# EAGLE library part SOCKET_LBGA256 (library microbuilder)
LBGA256 socket ... pitch is 1 mm
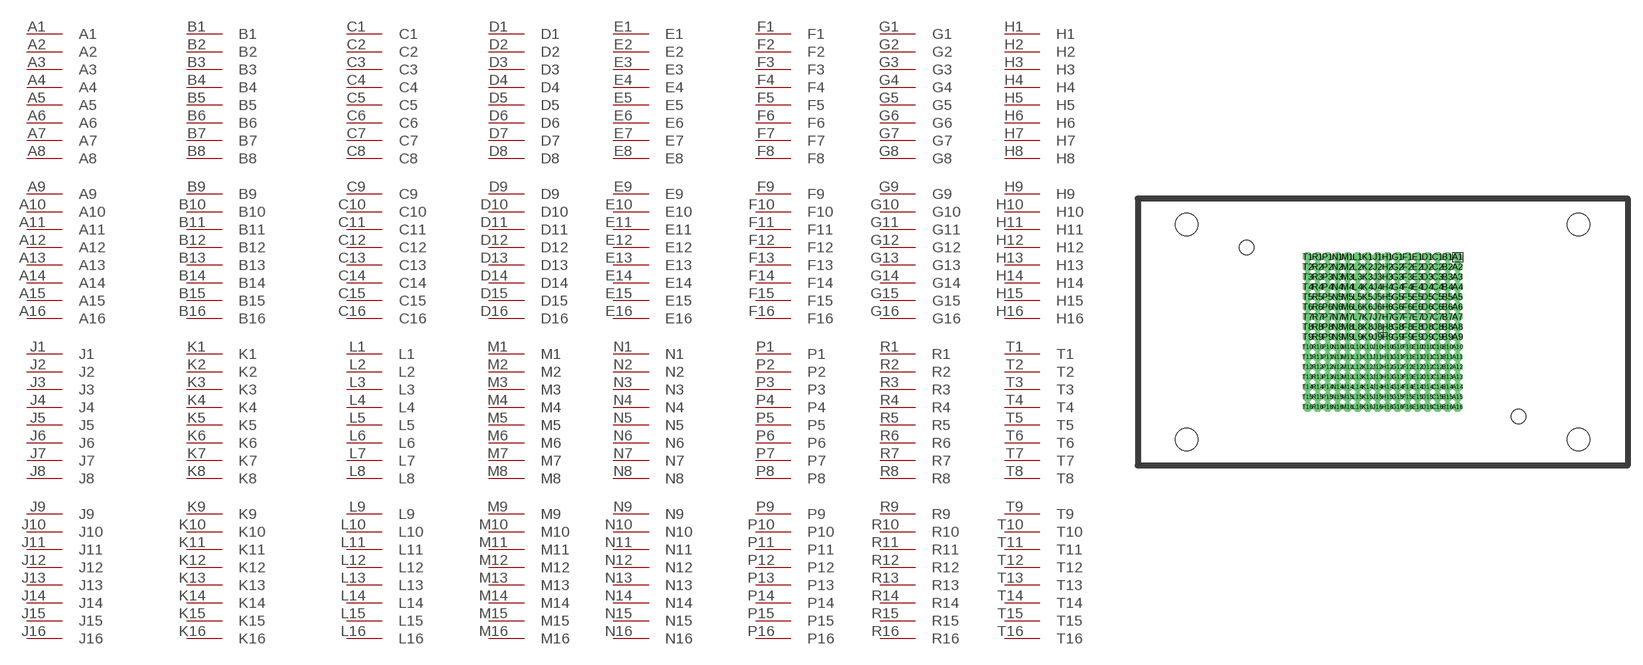
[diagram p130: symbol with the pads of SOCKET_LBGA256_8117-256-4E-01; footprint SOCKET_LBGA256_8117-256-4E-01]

Designator prefix IC

## SOCKET_LBGA256  [SOCKET_LBGA256_8117-256-4E-01]
A1  A1
A2  A2
A3  A3
A4  A4
A5  A5
A6  A6
A7  A7
A8  A8
A9  A9
A10  A10
A11  A11
A12  A12
A13  A13
A14  A14
A15  A15
A16  A16
B1  B1
B2  B2
B3  B3
B4  B4
B5  B5
B6  B6
B7  B7
B8  B8
B9  B9
B10  B10
B11  B11
B12  B12
B13  B13
B14  B14
B15  B15
B16  B16
C1  C1
C2  C2
C3  C3
C4  C4
C5  C5
C6  C6
C7  C7
C8  C8
C9  C9
C10  C10
C11  C11
C12  C12
C13  C13
C14  C14
C15  C15
C16  C16
D1  D1
D2  D2
D3  D3
D4  D4
D5  D5
D6  D6
D7  D7
D8  D8
D9  D9
D10  D10
D11  D11
D12  D12
D13  D13
D14  D14
D15  D15
D16  D16
E1  E1
E2  E2
E3  E3
E4  E4
E5  E5
E6  E6
E7  E7
E8  E8
E9  E9
E10  E10
E11  E11
E12  E12
E13  E13
E14  E14
E15  E15
E16  E16
F1  F1
F2  F2
F3  F3
F4  F4
F5  F5
F6  F6
F7  F7
F8  F8
F9  F9
F10  F10
F11  F11
F12  F12
F13  F13
F14  F14
F15  F15
F16  F16
G1  G1
G2  G2
G3  G3
G4  G4
G5  G5
G6  G6
G7  G7
G8  G8
G9  G9
G10  G10
G11  G11
G12  G12
G13  G13
G14  G14
G15  G15
G16  G16
H1  H1
H2  H2
H3  H3
H4  H4
H5  H5
H6  H6
H7  H7
H8  H8
H9  H9
H10  H10
H11  H11
H12  H12
H13  H13
H14  H14
H15  H15
H16  H16
J1  J1
J2  J2
J3  J3
J4  J4
J5  J5
J6  J6
J7  J7
J8  J8
J9  J9
J10  J10
J11  J11
J12  J12
J13  J13
J14  J14
J15  J15
J16  J16
K1  K1
K2  K2
K3  K3
K4  K4
K5  K5
K6  K6
K7  K7
K8  K8
K9  K9
K10  K10
K11  K11
K12  K12
K13  K13
K14  K14
K15  K15
K16  K16
L1  L1
L2  L2
L3  L3
L4  L4
L5  L5
L6  L6
L7  L7
L8  L8
L9  L9
L10  L10
L11  L11
L12  L12
L13  L13
L14  L14
L15  L15
L16  L16
M1  M1
M2  M2
M3  M3
M4  M4
M5  M5
M6  M6
M7  M7
M8  M8
M9  M9
M10  M10
M11  M11
M12  M12
M13  M13
M14  M14
M15  M15
M16  M16
N1  N1
N2  N2
N3  N3
N4  N4
N5  N5
N6  N6
N7  N7
N8  N8
N9  N9
N10  N10
N11  N11
N12  N12
N13  N13
N14  N14
N15  N15
N16  N16
P1  P1
P2  P2
P3  P3
P4  P4
P5  P5
P6  P6
P7  P7
P8  P8
P9  P9
P10  P10
P11  P11
P12  P12
P13  P13
P14  P14
P15  P15
P16  P16
R1  R1
R2  R2
R3  R3
R4  R4
R5  R5
R6  R6
R7  R7
R8  R8
R9  R9
R10  R10
R11  R11
R12  R12
R13  R13
R14  R14
R15  R15
R16  R16
T1  T1
T2  T2
T3  T3
T4  T4
T5  T5
T6  T6
T7  T7
T8  T8
T9  T9
T10  T10
T11  T11
T12  T12
T13  T13
T14  T14
T15  T15
T16  T16

## Footprint SOCKET_LBGA256_8117-256-4E-01 (pad centres in mm)
Wells 8117-256-4E-01 LBGA 256 socket LBGA256 ... pitch is 1 mm / diameter pin = 0.43 mm
drill 0.43 pad 0.7 octagon: A1 7.5,7.5; A2 7.5,6.5; A3 7.5,5.5; A4 7.5,4.5; A5 7.5,3.5; A6 7.5,2.5; A7 7.5,1.5; A8 7.5,0.5; A9 7.5,-0.5; A10 7.5,-1.5; A11 7.5,-2.5; A12 7.5,-3.5; A13 7.5,-4.5; A14 7.5,-5.5; A15 7.5,-6.5; A16 7.5,-7.5; B1 6.5,7.5; B2 6.5,6.5; B3 6.5,5.5; B4 6.5,4.5; B5 6.5,3.5; B6 6.5,2.5; B7 6.5,1.5; B8 6.5,0.5; B9 6.5,-0.5; B10 6.5,-1.5; B11 6.5,-2.5; B12 6.5,-3.5; B13 6.5,-4.5; B14 6.5,-5.5; B15 6.5,-6.5; B16 6.5,-7.5; C1 5.5,7.5; C2 5.5,6.5; C3 5.5,5.5; C4 5.5,4.5; C5 5.5,3.5; C6 5.5,2.5; C7 5.5,1.5; C8 5.5,0.5; C9 5.5,-0.5; C10 5.5,-1.5; C11 5.5,-2.5; C12 5.5,-3.5; C13 5.5,-4.5; C14 5.5,-5.5; C15 5.5,-6.5; C16 5.5,-7.5; D1 4.5,7.5; D2 4.5,6.5; D3 4.5,5.5; D4 4.5,4.5; D5 4.5,3.5; D6 4.5,2.5; D7 4.5,1.5; D8 4.5,0.5; D9 4.5,-0.5; D10 4.5,-1.5; D11 4.5,-2.5; D12 4.5,-3.5; D13 4.5,-4.5; D14 4.5,-5.5; D15 4.5,-6.5; D16 4.5,-7.5; E1 3.5,7.5; E2 3.5,6.5; E3 3.5,5.5; E4 3.5,4.5; E5 3.5,3.5; E6 3.5,2.5; E7 3.5,1.5; E8 3.5,0.5; E9 3.5,-0.5; E10 3.5,-1.5; E11 3.5,-2.5; E12 3.5,-3.5; E13 3.5,-4.5; E14 3.5,-5.5; E15 3.5,-6.5; E16 3.5,-7.5; F1 2.5,7.5; F2 2.5,6.5; F3 2.5,5.5; F4 2.5,4.5; F5 2.5,3.5; F6 2.5,2.5; F7 2.5,1.5; F8 2.5,0.5; F9 2.5,-0.5; F10 2.5,-1.5; F11 2.5,-2.5; F12 2.5,-3.5; F13 2.5,-4.5; F14 2.5,-5.5; F15 2.5,-6.5; F16 2.5,-7.5; G1 1.5,7.5; G2 1.5,6.5; G3 1.5,5.5; G4 1.5,4.5; G5 1.5,3.5; G6 1.5,2.5; G7 1.5,1.5; G8 1.5,0.5; G9 1.5,-0.5; G10 1.5,-1.5; G11 1.5,-2.5; G12 1.5,-3.5; G13 1.5,-4.5; G14 1.5,-5.5; G15 1.5,-6.5; G16 1.5,-7.5; H1 0.5,7.5; H2 0.5,6.5; H3 0.5,5.5; H4 0.5,4.5; H5 0.5,3.5; H6 0.5,2.5; H7 0.5,1.5; H8 0.5,0.5; H9 0.5,-0.5; H10 0.5,-1.5; H11 0.5,-2.5; H12 0.5,-3.5; H13 0.5,-4.5; H14 0.5,-5.5; H15 0.5,-6.5; H16 0.5,-7.5; J1 -0.5,7.5; J2 -0.5,6.5; J3 -0.5,5.5; J4 -0.5,4.5; J5 -0.5,3.5; J6 -0.5,2.5; J7 -0.5,1.5; J8 -0.5,0.5; J9 -0.5,-0.5; J10 -0.5,-1.5; J11 -0.5,-2.5; J12 -0.5,-3.5; J13 -0.5,-4.5; J14 -0.5,-5.5; J15 -0.5,-6.5; J16 -0.5,-7.5; K1 -1.5,7.5; K2 -1.5,6.5; K3 -1.5,5.5; K4 -1.5,4.5; K5 -1.5,3.5; K6 -1.5,2.5; K7 -1.5,1.5; K8 -1.5,0.5; K9 -1.5,-0.5; K10 -1.5,-1.5; K11 -1.5,-2.5; K12 -1.5,-3.5; K13 -1.5,-4.5; K14 -1.5,-5.5; K15 -1.5,-6.5; K16 -1.5,-7.5; L1 -2.5,7.5; L2 -2.5,6.5; L3 -2.5,5.5; L4 -2.5,4.5; L5 -2.5,3.5; L6 -2.5,2.5; L7 -2.5,1.5; L8 -2.5,0.5; L9 -2.5,-0.5; L10 -2.5,-1.5; L11 -2.5,-2.5; L12 -2.5,-3.5; L13 -2.5,-4.5; L14 -2.5,-5.5; L15 -2.5,-6.5; L16 -2.5,-7.5; M1 -3.5,7.5; M2 -3.5,6.5; M3 -3.5,5.5; M4 -3.5,4.5; M5 -3.5,3.5; M6 -3.5,2.5; M7 -3.5,1.5; M8 -3.5,0.5; M9 -3.5,-0.5; M10 -3.5,-1.5; M11 -3.5,-2.5; M12 -3.5,-3.5; M13 -3.5,-4.5; M14 -3.5,-5.5; M15 -3.5,-6.5; M16 -3.5,-7.5; N1 -4.5,7.5; N2 -4.5,6.5; N3 -4.5,5.5; N4 -4.5,4.5; N5 -4.5,3.5; N6 -4.5,2.5; N7 -4.5,1.5; N8 -4.5,0.5; N9 -4.5,-0.5; N10 -4.5,-1.5; N11 -4.5,-2.5; N12 -4.5,-3.5; N13 -4.5,-4.5; N14 -4.5,-5.5; N15 -4.5,-6.5; N16 -4.5,-7.5; P1 -5.5,7.5; P2 -5.5,6.5; P3 -5.5,5.5; P4 -5.5,4.5; P5 -5.5,3.5; P6 -5.5,2.5; P7 -5.5,1.5; P8 -5.5,0.5; P9 -5.5,-0.5; P10 -5.5,-1.5; P11 -5.5,-2.5; P12 -5.5,-3.5; P13 -5.5,-4.5; P14 -5.5,-5.5; P15 -5.5,-6.5; P16 -5.5,-7.5; R1 -6.5,7.5; R2 -6.5,6.5; R3 -6.5,5.5; R4 -6.5,4.5; R5 -6.5,3.5; R6 -6.5,2.5; R7 -6.5,1.5; R8 -6.5,0.5; R9 -6.5,-0.5; R10 -6.5,-1.5; R11 -6.5,-2.5; R12 -6.5,-3.5; R13 -6.5,-4.5; R14 -6.5,-5.5; R15 -6.5,-6.5; R16 -6.5,-7.5; T1 -7.5,7.5; T2 -7.5,6.5; T3 -7.5,5.5; T4 -7.5,4.5; T5 -7.5,3.5; T6 -7.5,2.5; T7 -7.5,1.5; T8 -7.5,0.5; T9 -7.5,-0.5; T10 -7.5,-1.5; T11 -7.5,-2.5; T12 -7.5,-3.5; T13 -7.5,-4.5; T14 -7.5,-5.5; T15 -7.5,-6.5; T16 -7.5,-7.5
hole 1.47 at 13.6,-8.45
hole 1.47 at -13.6,8.45
hole 2.26 at -19.6,10.75
hole 2.26 at -19.6,-10.75
hole 2.26 at 19.6,-10.75
hole 2.26 at 19.6,10.75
